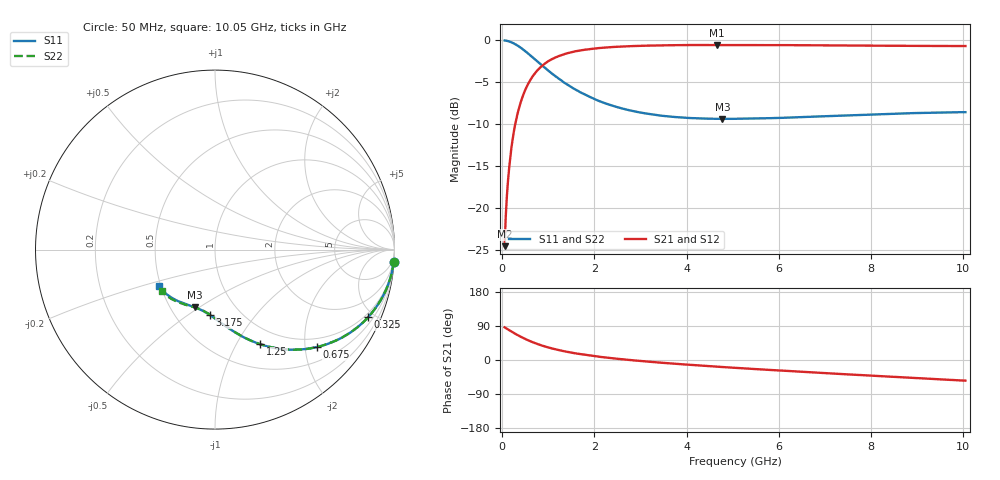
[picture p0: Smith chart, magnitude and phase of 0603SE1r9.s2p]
! AVX Thin Film Operation		Date: August 2001
! Description: Accu-P® Series, Thin Film, SMD, RF Capacitor
! Part Number: 06035J1R9ABT
! 50 MHz  -  10.05 GHz
! Serial Measurements
# mhz S db R 50
!	S11		S21		S12		S22
!	dB	Phase	dB	Phase	dB	Phase	dB	Phase
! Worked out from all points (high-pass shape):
!   401 points, 50 MHz to 10.05 GHz, reference 50 ohm
!   highest |S21| = -0.55 dB at 4.65 GHz (marker M1); lowest = -24.5 dB at 50 MHz (marker M2)
!   |S21| within 3 dB of the highest: 765.9 MHz to end of sweep
!   lowest |S11| = -9.4 dB at 4.775 GHz (marker M3), VSWR 2.03, Z = 33 - j24.1 ohm
!   |S11| at or under -10 dB: nowhere
!   |S22| runs from -9.3 to 0.0 dB; largest |S21 - S12| = 0
!   S11 on the Smith chart (normalised r, x): 50 MHz: 1, -30; 325 MHz: 0.80, -4.61; 675 MHz: 0.79, -2.25; 1.25 GHz: 0.79, -1.26; 3.175 GHz: 0.73, -0.61; 10.05 GHz: 0.49, -0.23
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50  -0.02 -3.8  -24.50 86.2  -24.50 86.2  -0.02 -3.8
75  -0.04 -5.7  -20.96 84.2  -20.96 84.2  -0.04 -5.7
125  -0.10 -9.5  -16.62 80.5  -16.62 80.5  -0.10 -9.5
175  -0.18 -13.2  -13.85 76.8  -13.85 76.8  -0.18 -13.2
250  -0.37 -18.6  -10.88 71.4  -10.88 71.4  -0.37 -18.6
325  -0.60 -23.8  -8.87 66.2  -8.87 66.2  -0.60 -23.8
475  -1.19 -33.2  -6.21 56.8  -6.21 56.8  -1.19 -33.2
675  -2.10 -43.8  -4.16 46.2  -4.16 46.2  -2.10 -43.8
825  -2.81 -50.4  -3.22 39.5  -3.22 39.5  -2.81 -50.4
975  -3.50 -56.1  -2.57 33.9  -2.57 33.9  -3.50 -56.0
1250  -4.66 -64.4  -1.82 25.6  -1.82 25.6  -4.66 -64.3
1450  -5.40 -69.4  -1.48 20.6  -1.48 20.6  -5.40 -69.3
1725  -6.27 -75.0  -1.18 15.0  -1.18 15.0  -6.27 -74.9
2325  -7.66 -84.6  -0.82 5.4  -0.82 5.4  -7.66 -84.3
3175  -8.76 -94.5  -0.63 -4.4  -0.63 -4.4  -8.76 -94.0
3400  -8.93 -97.0  -0.60 -6.7  -0.60 -6.7  -8.93 -96.2
4650  -9.34 -108.1  -0.55 -17.6  -0.55 -17.6  -9.33 -106.1
4775  -9.35 -109.0  -0.55 -18.5  -0.55 -18.5  -9.33 -107.1
5050  -9.34 -111.0  -0.55 -20.7  -0.55 -20.7  -9.33 -110.0
6725  -9.09 -124.0  -0.59 -32.7  -0.59 -32.7  -9.07 -121.0
8400  -8.75 -136.1  -0.65 -43.9  -0.65 -43.9  -8.72 -131.2
10050  -8.55 -146.8  -0.68 -54.4  -0.68 -54.4  -8.52 -141.6
